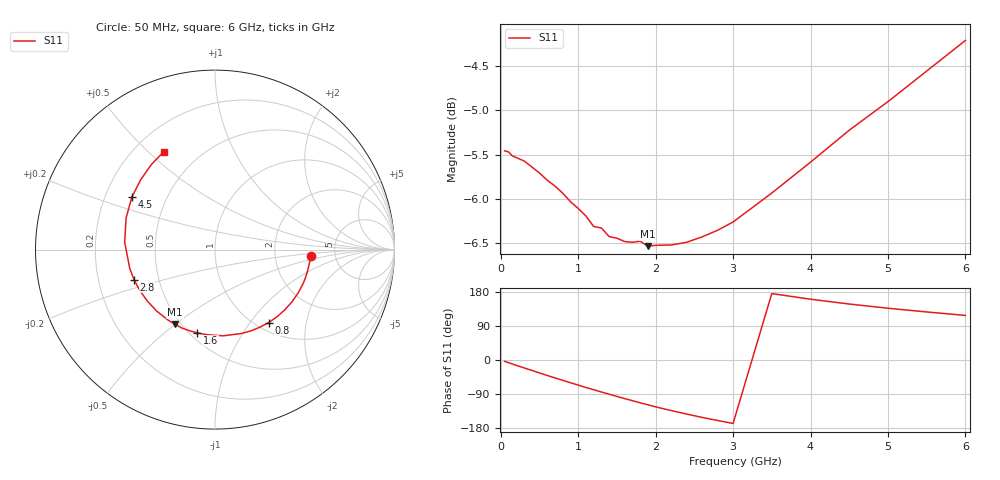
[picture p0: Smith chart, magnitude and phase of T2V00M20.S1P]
! SIEMENS Discrete & RF Semiconductors
! BAS70-04W
! Si Schottky Diode in SOT323
! IF = 0.2 mA
! S-Parameters:  November  1997
# GHz  S  MA  R  50
!  f  S11
! GHz  MAG  ANG
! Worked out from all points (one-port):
!   34 points, 50 MHz to 6 GHz, reference 50 ohm
!   lowest |S11| = -6.5 dB at 1.9 GHz (marker M1), VSWR 2.78, Z = 23.3 - j24.9 ohm
!   |S11| at or under -10 dB: nowhere
!   S11 on the Smith chart (normalised r, x): 50 MHz: 3.26, -0.30; 800 MHz: 1.14, -1.24; 1.6 GHz: 0.55, -0.65; 2.8 GHz: 0.36, -0.16; 4.5 GHz: 0.31, +0.26; 6 GHz: 0.32, +0.56
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0.05  0.5335 -3.6
0.1  0.5328 -7.0
0.25  0.5277 -17.3
0.4  0.5225 -27.4
0.5  0.5183 -34.1
0.6  0.5135 -40.8
0.7  0.5096 -47.2
0.8  0.505 -53.6
0.9  0.4994 -60.0
1  0.495 -66.2
1.1  0.4902 -72.6
1.3  0.4826 -84.5
1.5  0.4762 -96.0
1.6  0.4742 -101.9
1.8  0.4744 -113.0
1.9  0.4713 -118.2
2  0.4719 -123.6
2.2  0.472 -133.4
2.4  0.4737 -142.6
2.6  0.477 -151.5
2.8  0.4812 -159.6
3  0.4864 -167.5
3.5  0.505 175.3
4  0.5257 160.4
4.5  0.548 147.7
5  0.5687 136.6
5.5  0.5918 126.8
6  0.6158 117.6
